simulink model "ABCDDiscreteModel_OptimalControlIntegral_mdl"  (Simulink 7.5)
settings: Solver=FixedStepDiscrete  StartTime=0.0  StopTime=10.0  FixedStep=Ts  RelTol=1e-3
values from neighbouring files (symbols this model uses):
  H = Ki(n+1)    [TSC140415ProvaMatlab.m]
  K = Ki(1:n)    [TSC140415ProvaMatlab.m]
  tp = 2    [TSC140415ProvaMatlab.m]
  Ts = 0.05    [TSC140415ProvaMatlab.m]
  X0 = [0 0 0.5]    [TSC140415ProvaMatlab.m]
  yp = 4    [TSC140415ProvaMatlab.m]
undefined symbols (not defined in the file or in its folder): A, B, C, D, DiscIntNeverNeededParam

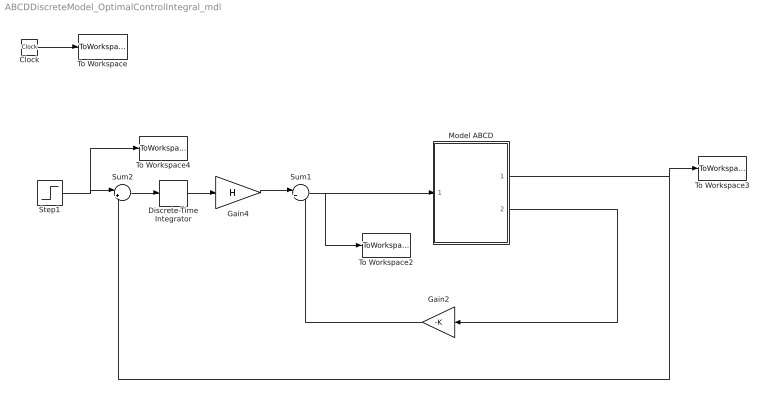
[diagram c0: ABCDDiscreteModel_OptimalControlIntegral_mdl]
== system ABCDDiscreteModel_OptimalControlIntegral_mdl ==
  Clock : Clock
  Discrete-Time Integrator : DiscreteIntegrator  SampleTime=Ts  OutDataType=sfix(16)  OutScaling=2^0  ICPrevOutput=DiscIntNeverNeededParam  ICPrevScaledInput=DiscIntNeverNeededParam
  Gain2 : Gain  Gain=-K  Multiplication=Matrix(K*u)  ParameterDataType=sfix(16)  ParameterScaling=2^0  OutDataType=sfix(16)  OutScaling=2^0
  Gain4 : Gain  Gain=H  Multiplication=Matrix(K*u)  ParameterDataType=sfix(16)  ParameterScaling=2^0  OutDataType=sfix(16)  OutScaling=2^0
  Model ABCD : Subsystem
  Step1 : Step  Time=tp  After=yp  SampleTime=0
  Sum1 : Sum  Inputs=|++  OutDataType=sfix(16)  OutScaling=2^0
  Sum2 : Sum  Inputs=|+-  OutDataType=sfix(16)  OutScaling=2^0
  To Workspace : ToWorkspace  VariableName=time  SampleTime=-1  SaveFormat=Array
  To Workspace2 : ToWorkspace  VariableName=u  SampleTime=-1  SaveFormat=Array
  To Workspace3 : ToWorkspace  VariableName=y  SampleTime=-1  SaveFormat=Array
  To Workspace4 : ToWorkspace  VariableName=yd  SampleTime=-1  SaveFormat=Array
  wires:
  Gain4/1 -> Sum1/1
  Step1/1 -> To Workspace4/1, Sum2/1
  Gain2/1 -> Sum1/2
  Sum1/1 -> To Workspace2/1, Model ABCD/1(U)
  Model ABCD/2(X) -> Gain2/1
  Clock/1 -> To Workspace/1
  Model ABCD/1(Y) -> To Workspace3/1, Sum2/2
  Discrete-Time Integrator/1 -> Gain4/1
  Sum2/1 -> Discrete-Time Integrator/1

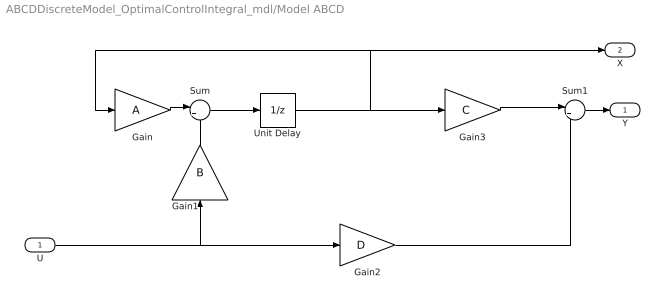
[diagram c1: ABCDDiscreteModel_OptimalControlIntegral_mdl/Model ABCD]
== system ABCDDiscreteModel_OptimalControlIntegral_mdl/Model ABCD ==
  U : Inport
  Gain : Gain  Gain=A  Multiplication=Matrix(K*u)  ParameterDataType=sfix(16)  ParameterScaling=2^0  OutDataType=sfix(16)  OutScaling=2^0
  Gain1 : Gain  Gain=B  Multiplication=Matrix(K*u)  ParameterDataType=sfix(16)  ParameterScaling=2^0  OutDataType=sfix(16)  OutScaling=2^0
  Gain2 : Gain  Gain=D  Multiplication=Matrix(K*u)  ParameterDataType=sfix(16)  ParameterScaling=2^0  OutDataType=sfix(16)  OutScaling=2^0
  Gain3 : Gain  Gain=C  Multiplication=Matrix(K*u)  ParameterDataType=sfix(16)  ParameterScaling=2^0  OutDataType=sfix(16)  OutScaling=2^0
  Sum : Sum  Inputs=|++  OutDataType=sfix(16)  OutScaling=2^0
  Sum1 : Sum  Inputs=|++  OutDataType=sfix(16)  OutScaling=2^0
  Unit Delay : UnitDelay  X0=X0  SampleTime=Ts
  Y : Outport
  X : Outport  Port=2
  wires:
  Gain/1 -> Sum/1
  Gain1/1 -> Sum/2
  Sum/1 -> Unit Delay/1
  Unit Delay/1 -> Gain3/1, Gain/1, X/1
  Gain3/1 -> Sum1/1
  U/1 -> Gain1/1, Gain2/1
  Gain2/1 -> Sum1/2
  Sum1/1 -> Y/1
